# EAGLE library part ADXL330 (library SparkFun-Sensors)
Analog Devices ADXL330 3-Axis Analog Accelerometer The ADXL330 is a small, thin, low power, complete 3-axis accelerometer with signal conditioned voltage outputs, all on a single monolithic IC. The product measures acceleration with a minimum full-scale range of ±3g. It can measure the static acceleration of gravity in tilt-sensing applications, as well as dynamic acceleration resulting from motion, shock, or vibration. Datasheet SparkFun Products Triple Axis Accelerometer Breakout - ADXL330 (SEN-00692)
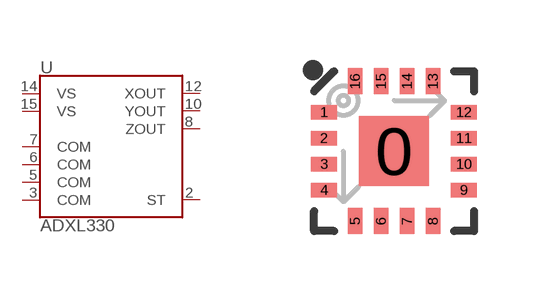
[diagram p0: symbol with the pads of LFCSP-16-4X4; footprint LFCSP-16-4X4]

Designator prefix U

## ADXL330 (PROD_ID: IC-08189)  [LFCSP-16-4X4]
2  ST
3  COM
5  COM
6  COM
7  COM
8  ZOUT
10  YOUT
12  XOUT
14  VS
15  VS

## Footprint LFCSP-16-4X4 (pad centres in mm)
16-Pin LFCSP w/ Center Pad (4 x 4 mm) Datasheet Specifications: Pin Count: 16 (+ center pad) Area: 4.0 x 4.0 x 1.45 mm Pitch: 0.65 mm Devices Using: ADXL330 ADXL335
smd 1.75 x 1.75: 0 0,0
smd 0.65 x 0.37: 1 -1.75,0.975; 2 -1.75,0.325; 3 -1.75,-0.325; 4 -1.75,-0.975; 9 1.75,-0.975; 10 1.75,-0.325; 11 1.75,0.325; 12 1.75,0.975
smd 0.37 x 0.65: 5 -0.975,-1.75; 6 -0.325,-1.75; 7 0.325,-1.75; 8 0.975,-1.75; 13 0.975,1.75; 14 0.325,1.75; 15 -0.325,1.75; 16 -0.975,1.75

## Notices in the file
Licensing: Creative Commons ShareAlike 4.0 International - https://creativecommons.org/licenses/by-sa/4.0
